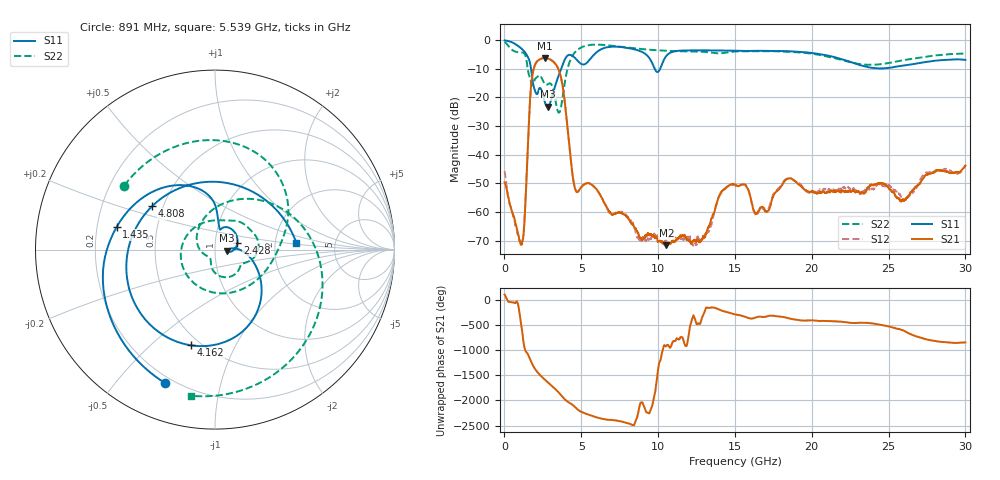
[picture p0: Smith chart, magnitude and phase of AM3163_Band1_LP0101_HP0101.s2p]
!Agilent Technologies,E8364B,MY43040894,A.07.50.67
!Agilent E8364B: A.07.50.67
!Date: Thursday, August 20, 2020 11:18:24
!Correction: S11(Full 2 Port(1,2))
!S21(Full 2 Port(1,2))
!S12(Full 2 Port(1,2))
!S22(Full 2 Port(1,2))
!S2P File: Measurements: S11, S21, S12, S22:
# Hz S  dB  R 50
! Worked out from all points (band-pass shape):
!   3201 points, 10 MHz to 30 GHz, reference 50 ohm
!   highest |S21| = -6.19 dB at 2.615 GHz (marker M1); lowest = -71.7 dB at 10.53 GHz (marker M2)
!   |S21| within 3 dB of the highest: 1.949 GHz to 3.432 GHz (1.483 GHz wide, 55.1 % of centre)
!   lowest |S11| = -23.3 dB at 2.812 GHz (marker M3), VSWR 1.15, Z = 57.3 - j0.782 ohm
!   |S11| at or under -10 dB: 1.732 GHz to 3.685 GHz (1.953 GHz wide, 72.1 % of centre); 9.779 GHz to 10.13 GHz (354 MHz wide, 3.56 % of centre)
!   |S22| runs from -25.3 to -0.6 dB; largest |S21 - S12| = 0.0067
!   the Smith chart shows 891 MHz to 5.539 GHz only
!   S11 on the Smith chart (normalised r, x): 891 MHz: 0.17, -0.68; 1.435 GHz: 0.28, +0.10; 2.428 GHz: 1.28, +0.09; 4.162 GHz: 0.44, -0.68; 4.808 GHz: 0.44, +0.26; 5.539 GHz: 2.64, +0.24
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1e7  -0.08 -7.9  -49.61 101.5  -45.66 0.9  -0.60 -24.6
4.879656e8  -0.72 -59.7  -59.87 -50.5  -59.76 -49.2  -3.33 -141.9
8.909562e8  -2.00 -110.4  -67.69 -100.3  -68.61 158.3  -4.17 144.8
1.434525e9  -5.00 167.0  -48.66 36.3  -48.17 54.8  -6.97 24.6
1.8094e9  -13.42 87.3  -12.47 161.2  -12.47 161.1  -15.66 121.8
2.427944e9  -17.77 15.9  -6.38 -89.5  -6.38 -89.6  -13.30 -13.6
2.615381e9  -21.38 -8.6  -6.19 -143.5  -6.20 -143.6  -15.20 -26.1
2.812191e9  -23.26 -5.7  -6.35 162.5  -6.36 162.5  -15.40 -34.9
3.561941e9  -11.81 -24.3  -10.79 -52.3  -10.80 -52.2  -25.28 -130.8
4.161741e9  -5.20 -104.1  -33.76 126.4  -33.71 126.5  -8.84 50.6
4.8084e9  -7.43 145.1  -52.74 -29.8  -52.83 -30.8  -3.13 -38.2
5.014581e9  -8.32 104.9  -51.17 -67.4  -51.28 -68.0  -2.47 -57.9
5.539406e9  -6.84 4.6  -50.07 -127.6  -50.15 -126.1  -1.67 -99.2
6.392247e9  -2.91 -95.5  -55.61 155.6  -55.74 151.2  -1.61 -150.7
7.460641e9  -2.31 -169.8  -60.22 112.7  -60.21 110.6  -2.19 158.9
1.000979e10  -10.99 96.6  -70.25 82.0  -68.81 63.0  -3.54 59.8
1.053462e10  -5.50 94.8  -71.66 160.8  -69.90 -133.0  -3.70 41.0
1.240899e10  -3.54 7.3  -70.14 -33.3  -71.18 -129.1  -3.96 -22.1
1.5005e10  -3.65 -72.1  -50.39 68.1  -50.71 67.3  -3.95 -90.2
2.000958e10  -4.44 163.4  -52.73 -50.1  -52.68 -53.3  -4.71 136.7
2.500479e10  -9.67 -62.3  -51.66 -170.8  -50.78 -171.1  -7.96 -92.1
3e10  -6.88 104.4  -43.80 -129.2  -43.81 -128.6  -4.63 102.6
